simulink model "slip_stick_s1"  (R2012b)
settings: Solver=ode2  StartTime=0.0  StopTime=100  FixedStep=0.001  MaxStep=0.001  RelTol=1e-3
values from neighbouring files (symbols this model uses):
  c = 2200    [coulomb_1.m]    (also in coulomb_10.m = 0.1; coulomb_11.m = 0; coulomb_2.m; coulomb_3.m)
  f = FG    (= 500)    [coulomb_5.m]    (also in dry_friction_1.m; feder_masse_1.m = logspace(e1,e2,5000); feder_masse_11.m = logspace(e1,e2,5000); feder_masse_12.m = logspace(e1,e2,5000))
  k = 10    [coulomb_10.m]    (also in coulomb_11.m; diff_filter_1.m = 250; diff_filter_2.m = 250; dry_friction_1.m = 2200)
  m = 400    [coulomb_1.m]    (also in coulomb_10.m = 10; coulomb_11.m = 10; coulomb_2.m; coulomb_3.m)
  vb = 0.1    [coulomb_10.m]    (also in coulomb_11.m; slip_stick_3.m; slip_stick_31.m; slip_stick_3_1.m)

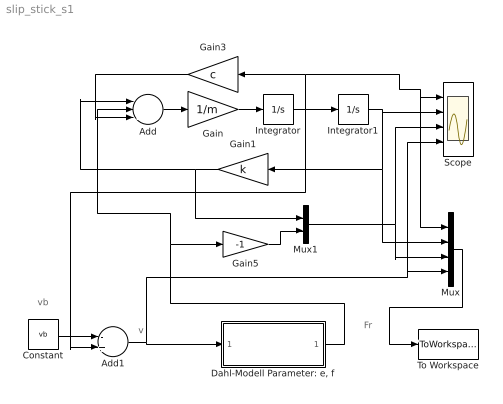
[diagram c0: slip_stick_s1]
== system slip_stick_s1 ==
  note: v
  note: vb
  note: Fr
  Add : Sum  Inputs=---
  Add1 : Sum  Inputs=-+
  Constant : Constant  Value=vb
  "Dahl-Modell Parameter: e, f" : Subsystem
  Gain : Gain  Gain=1/m
  Gain1 : Gain  Gain=k
  Gain3 : Gain  Gain=c
  Gain5 : Gain  Gain=-1
  Integrator : Integrator
  Integrator1 : Integrator
  Mux : Mux
  Mux1 : Mux  Inputs=2
  Scope : Scope  NumInputPorts=4
  To Workspace : ToWorkspace  VariableName=y  SampleTime=-1  SaveFormat=Structure With Time
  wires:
  Add/1 -> Gain/1
  Gain/1 -> Integrator/1
  Integrator1/1 -> Mux/2, Gain1/1, Scope/2
  Constant/1 -> Add1/1
  Integrator/1 -> Add1/2, Integrator1/1, Mux/1, Scope/1, Gain3/1
  Gain3/1 -> Add/3
  "Dahl-Modell Parameter: e, f"/1(Fr) -> Add/2, Gain5/1
  Gain1/1 -> Mux1/1, Add/1
  Mux1/1 -> Mux/3, Scope/3
  Gain5/1 -> Mux1/2
  Add1/1 -> Mux/4, Scope/4, "Dahl-Modell Parameter: e, f"/1(v)
  Mux/1 -> To Workspace/1

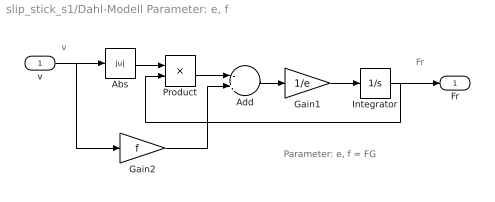
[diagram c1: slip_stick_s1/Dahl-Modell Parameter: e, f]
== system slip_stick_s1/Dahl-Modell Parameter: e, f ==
  note: v
  note: Fr
  note: Parameter: e, f = FG
  v : Inport
  Abs : Abs
  Add : Sum  Inputs=-+
  Gain1 : Gain  Gain=1/e
  Gain2 : Gain  Gain=f
  Integrator : Integrator
  Product : Product
  Fr : Outport
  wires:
  Integrator/1 -> Product/2, Fr/1
  Abs/1 -> Product/1
  Add/1 -> Gain1/1
  v/1 -> Abs/1, Gain2/1
  Product/1 -> Add/1
  Gain2/1 -> Add/2
  Gain1/1 -> Integrator/1
